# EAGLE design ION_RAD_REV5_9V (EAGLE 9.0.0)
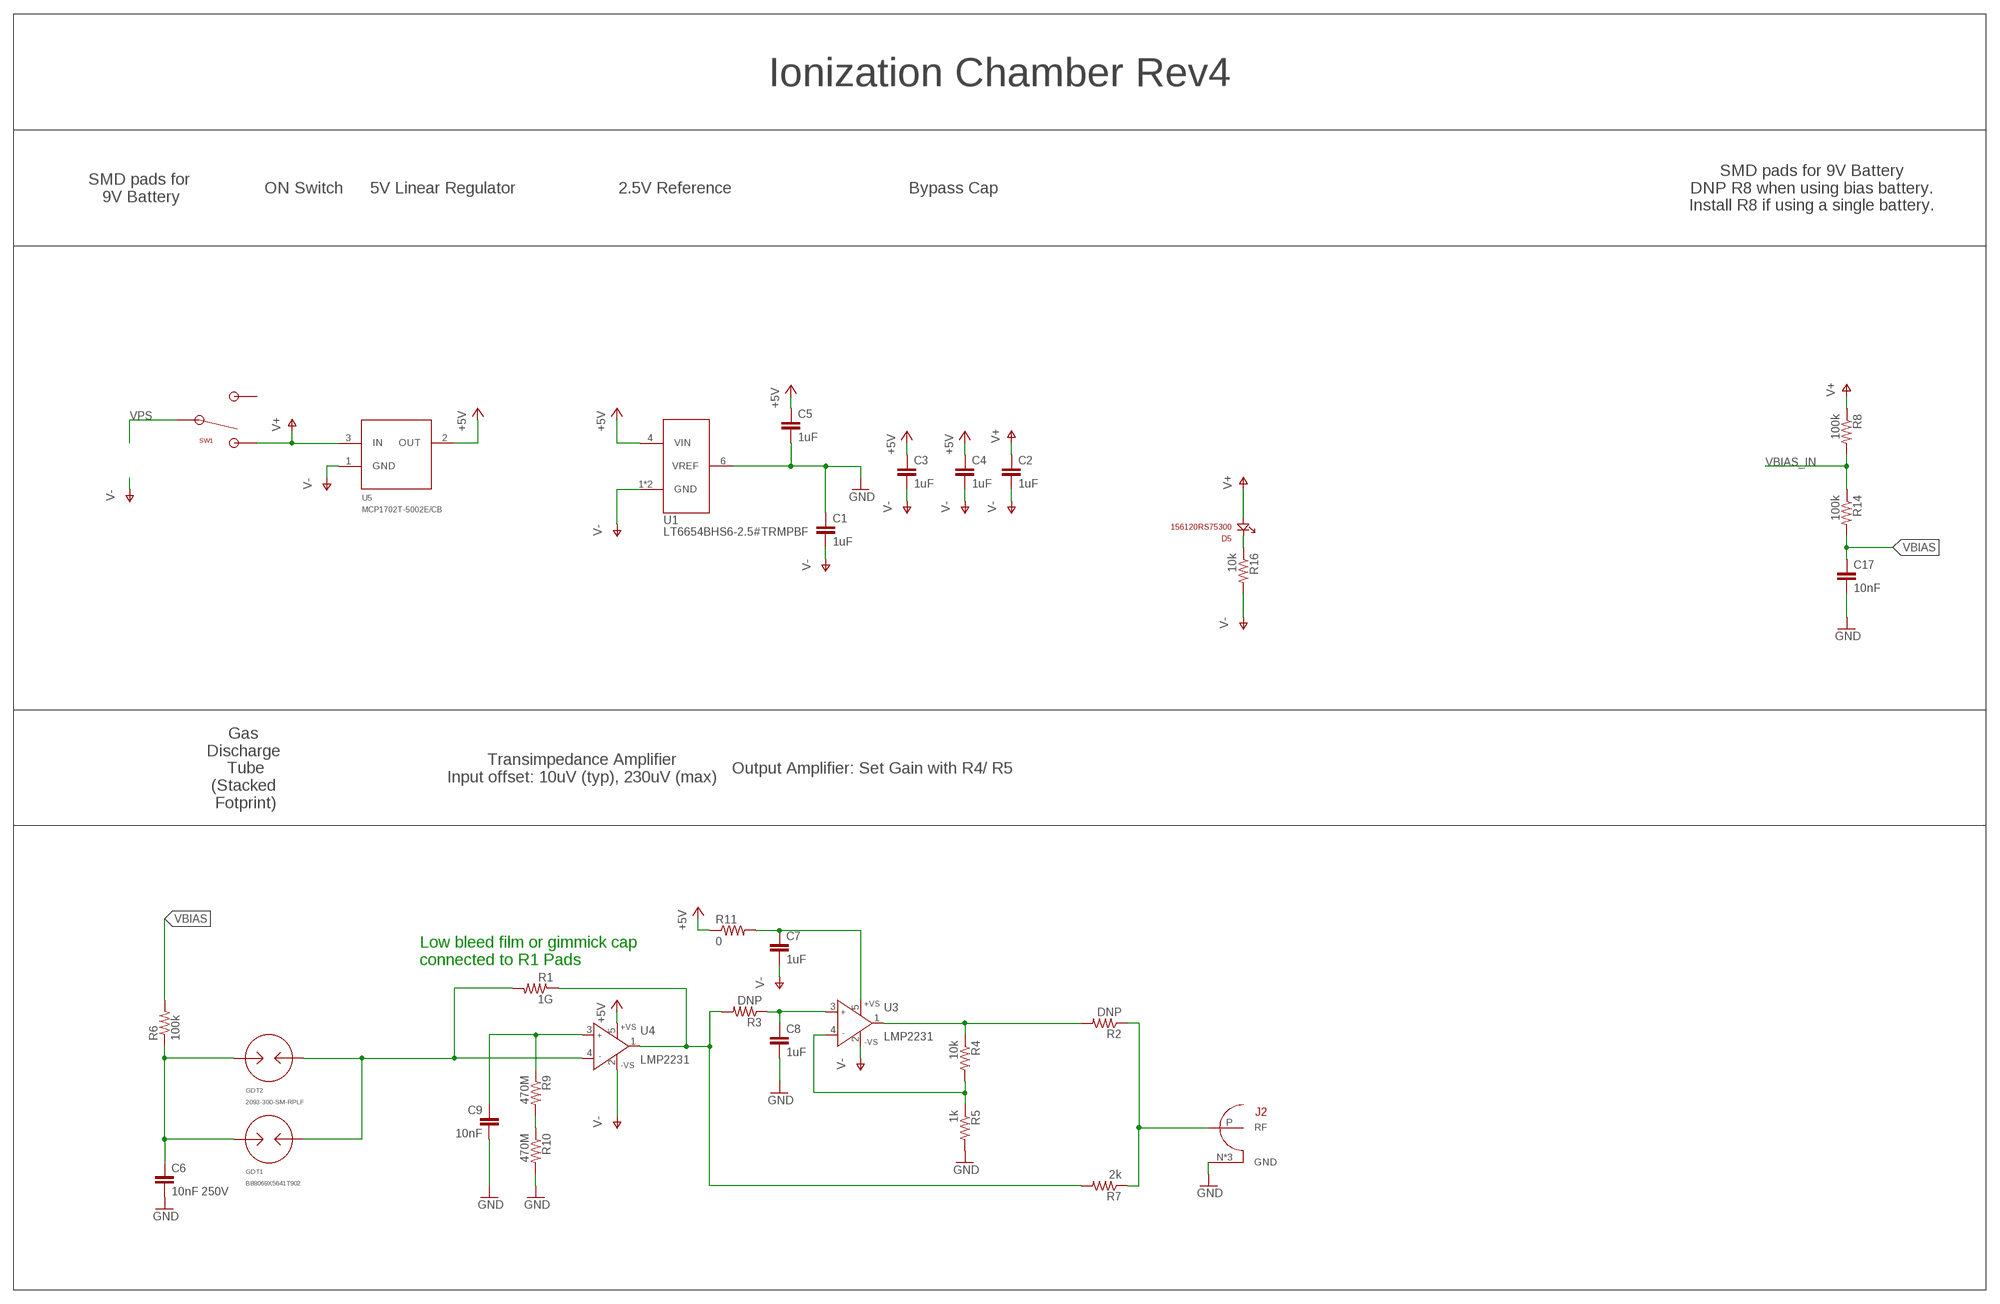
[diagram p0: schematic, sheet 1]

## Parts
C1  1uF  0805_CAPACITOR  [0805]
C2  1uF  0805_CAPACITOR  [0805]
C3  1uF  0805_CAPACITOR  [0805]
C4  1uF  0805_CAPACITOR  [0805]
C5  1uF  0805_CAPACITOR  [0805]
C6  10nF 250V  0805_CAPACITOR  [0805]
C7  1uF  0805_CAPACITOR  [0805]
C8  1uF  0805_CAPACITOR  [0805]
C9  10nF  0805_CAPACITOR  [0805]
C17  10nF  0805_CAPACITOR  [0805]
D5  156120RS75300  [1206_REV]
GDT1  B88069X5641T902  [ES1200XSMD]
GDT2  2093-300-SM-RPLF  [2093-300-SM-RPLF]
J2  0731385033  [0731385033]
R1  1G  MHR0317SA108F70  [MHR0317_SMD]
R2  DNP  0603_RESISTOR  [0603]
R3  DNP  0603_RESISTOR  [0603]
R4  10k  0603_RESISTOR  [0603]
R5  1k  0603_RESISTOR  [0603]
R6  100k  0603_RESISTOR  [0603]
R7  2k  0603_RESISTOR  [0603]
R8  100k  0603_RESISTOR  [0603]
R9  470M  0603_RESISTOR  [0603]
R10  470M  0603_RESISTOR  [0603]
R11  0  0603_RESISTOR  [0603]
R14  100k  0603_RESISTOR  [0603]
R16  10k  0603_RESISTOR  [0603]
SW1  SPDT  100SP1T2B4M6QE  [TOGGLE_RA]
U1  LT6654BHS6-2.5#TRMPBF  [SOT23-6]
U3  LMP2231  [SOT23-5]
U4  LMP2231  [SOT23-5]
U5  MCP1702T-5002E/CB  [SOT23-3_CENTERED]

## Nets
+5V: C3.1 C4.1 C5.1 R11.1 U1.4(VIN) U4.5(+VS) U5.2(OUT)
GND: C1.1 C5.2 C6.2 C8.2 C9.2 C17.2 J2.N(GND) J2.S1(GND) J2.S2(GND) R5.2 R10.2 U1.6(VREF)
INN: GDT1.P$2 GDT2.P$2 R1.P$2 U4.4(IN-)
N$1: C8.1 R3.1 U3.3(IN+)
N$2: R2.2 R4.1 U3.1(OUT)
N$3: R4.2 R5.1 U3.4(IN-)
N$4: C9.1 R9.1 U4.3(IN+)
N$5: J2.P(RF) R2.1 R7.1
N$6: R9.2 R10.1
N$7: C6.1 GDT1.P$1 GDT2.P$1 R6.1
N$10: C7.1 R11.2 U3.5(+VS)
N$19: D5.K R16.1
OUT: R1.P$1 R3.2 R7.2 U4.1(OUT)
V+: C2.1 D5.A R8.1 SW1.3 U5.3(IN)
V-: C1.2 C2.2 C3.2 C4.2 C7.2 R16.2 U1.1(GND) U1.2(GND) U3.2(-VS) U4.2(-VS) U5.1(GND)
VBIAS: C17.1 R6.2 R14.2
VBIAS_IN: R8.2 R14.1
VPS: SW1.2(COM)
Unconnected: SW1.1

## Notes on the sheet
- Ionization Chamber Rev4
- SMD pads for 
  9V Battery
- ON Switch | 5V Linear Regulator | 2.5V Reference | Bypass Cap
- SMD pads for 9V Battery
  DNP R8 when using bias battery.
  Install R8 if using a single battery.
- Gas 
  Discharge 
  Tube
  (Stacked 
  Fotprint)
- Transimpedance Amplifier
  Input offset: 10uV (typ), 230uV (max)
- Output Amplifier: Set Gain with R4/ R5
- Low bleed film or gimmick cap
  connected to R1 Pads

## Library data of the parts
C1-C9 C17 = ruark2:0805_CAPACITOR: NO DEFINED PN
D5 = ruark2:156120RS75300: Red 624nm LED Indication - Discrete 2V 1206 Reverse Mount (3216 Metric); PARTNO: 732-5031-1-ND
GDT1 = ruark2:B88069X5641T902: Gas Discharge Tube 1200V 1000A (1kA) ±15% 2 Pole Surface Mount; PARTNO: 495-76508-1-ND
GDT2 = ruark2:2093-300-SM-RPLF: Gas Discharge Tube 3000V 3000A (3kA) ±20% 2 Pole Surface Mount; PARTNO: 2093-300-SM-RPLFCT-ND
J2 = ruark2:0731385033: BNC Connector Jack, Female Socket 50Ohm Panel Mount, Through Hole, Right Angle Solder; PARTNO: WM5515-ND
R1 = ruark2:MHR0317SA108F70: 1 GOhms ±1% 0.8W Through Hole Resistor Radial High Voltage Thick Film; PARTNO: 490-18223-ND
R2-R11 R14 R16 = ruark2:0603_RESISTOR: 0603 Resistor -- WARNING: NO DEFINED PART NUMBER OR VALUE; VALUE: sel
SW1 = ruark2:100SP1T2B4M6QE: Toggle Switch SPDT Through Hole, Right Angle 5A 120V; PARTNO: EG2362-ND
U1 = ruark2:LT6654BHS6-2.5#TRMPBF: 2.5V Series Voltage Reference IC ±0.1% TSOT-23-6; PARTNO: LT6654BHS6-2.5#TRMPBFCT-ND
U3 U4 = ruark2:LMP2231: General Purpose Amplifier 1 Circuit Rail-to-Rail SOT-23-5, 0.02pA, 10uV
U5 = ruark2:MCP1702T-5002E/CB: Linear Voltage Regulator IC Positive Fixed 1 Output 250mA SOT-23A-3; PARTNO: MCP1702T-5002E/CBCT-ND

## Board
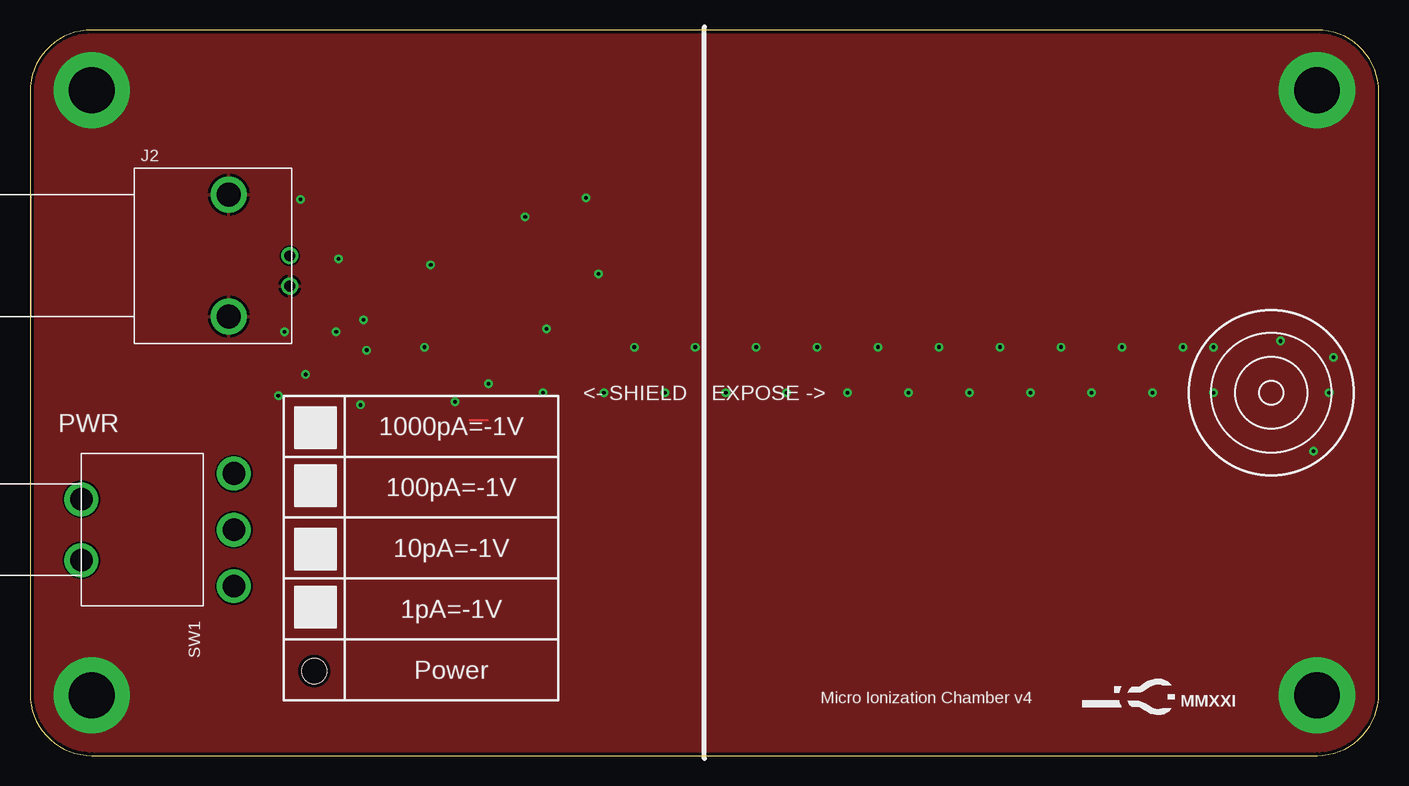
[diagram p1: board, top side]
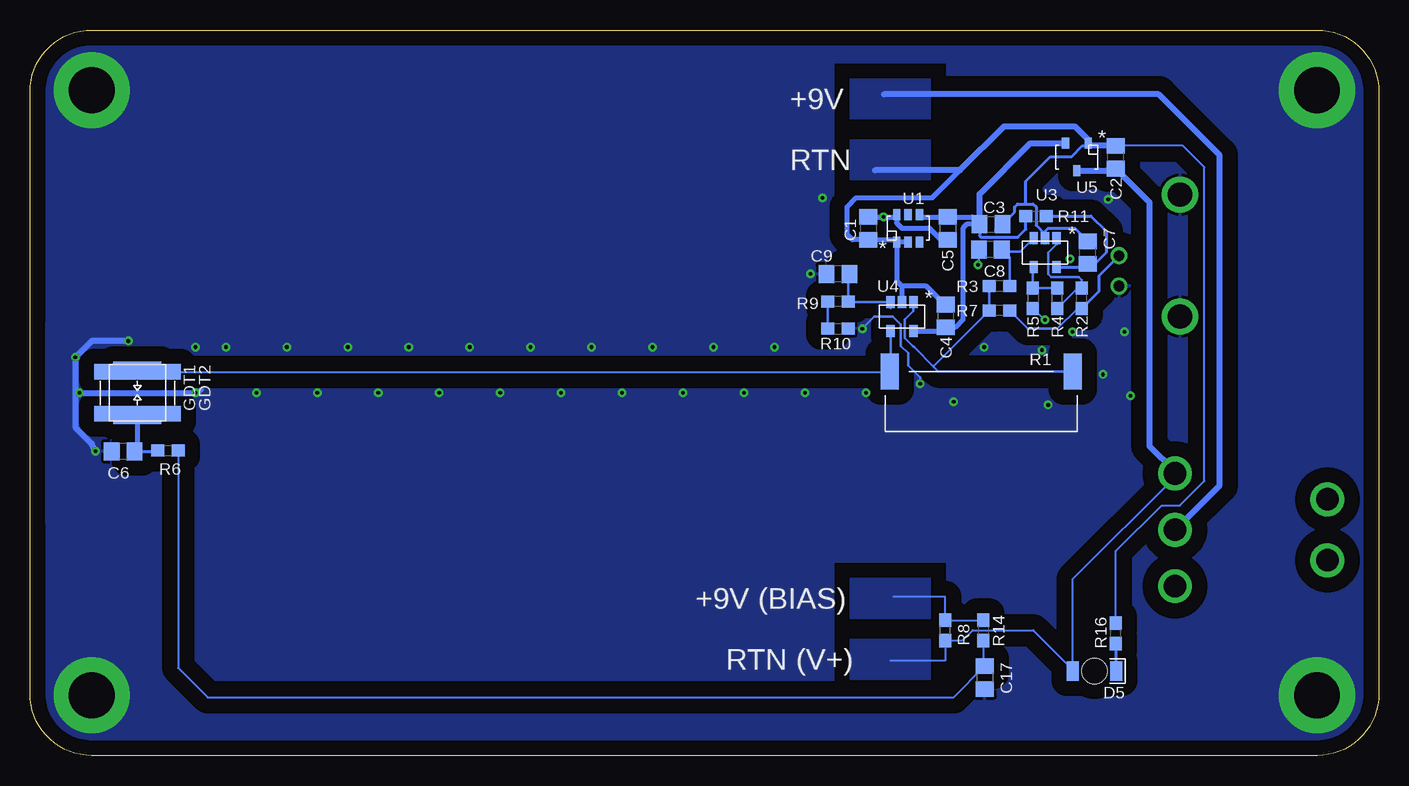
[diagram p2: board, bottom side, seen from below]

Size 112.4 x 60.5 mm. Coordinates in mm from the lower left corner, seen from the top.
Outline: 0,55.35 0,5.15 arc90 5.15,0 107.25,0 arc90 112.4,5.15 112.4,55.35 arc90 107.25,60.5 5.15,60.5 arc90 0,55.35
Copper layers (1*16): Top 0.035mm / dielectric 1.5mm / Bottom 0.035mm
Design rules "default *": minimum track width 6mil, minimum drill 12mil, track to track 6mil, track to pad 6mil, pad to pad 6mil, via to via 6mil, smd to smd 6mil, copper to edge 0.3mm, drill to drill 6mil, minimum pad ring 10mil, minimum via ring 8mil, stop-mask expansion 4mil, vias tented up to drill 12mil, thermal gap 10mil

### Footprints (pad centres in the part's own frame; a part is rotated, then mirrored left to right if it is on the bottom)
0805 = smd 1.3 x 1.5: 1 -0.95,0; 2 0.95,0
1206_REV = smd 1 x 1.6: A -1.8,0; K 1.8,0 | hole 2.1: 0,0
ES1200XSMD = smd 1.25 x 4: P$1 -1.975,0; P$2 1.975,0
2093-300-SM-RPLF = smd 1.3 x 7.2: P$1 -1.75,0; P$2 1.75,0
0731385033 = drill 0.889: N -2.54,-5.08; P 0,-5.08 | drill 2.007: S1 -5.08,0; S2 5.08,0
MHR0317_SMD = smd 1.5 x 3: P$1 -7.62,0; P$2 7.62,0
0603 = smd 1.1 x 1: 1 -0.85,0; 2 0.85,0
TOGGLE_RA = drill 1.88: 1 4.699,12.7; 2 0,12.7; 3 -4.699,12.7; P$4 -2.54,0; P$5 2.54,0
SOT23-6 = smd 0.6 x 0.9: 1 -0.95,-1.15; 2 0,-1.15; 3 0.95,-1.15; 4 0.95,1.15; 5 0,1.15; 6 -0.95,1.15
SOT23-5 = smd 0.7 x 1: 1 0.95,1.2; 2 0,1.2; 3 -0.95,1.2; 4 -0.95,-1.2; 5 0.95,-1.2
SOT23-3_CENTERED = smd 0.6 x 0.9: 1 -0.95,-1.15; 2 0.95,-1.15; 3 0,1.15

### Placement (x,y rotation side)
C1  42.53,43.97 270 bottom
C2  21.91,49.88 90 bottom
C3  32.32,44.3 0 bottom
C4  36.07,36.65 90 bottom
C5  35.93,43.97 270 bottom
C6  104.63,25.36 180 bottom
C7  24.25,41.93 90 bottom
C8  32.37,42.19 180 bottom
C9  45.07,40.16 180 bottom
C17  32.83,6.5 270 bottom
D5  23.69,7.03 0 bottom
GDT1  103.44,30.25 90 bottom
GDT2  103.44,30.25 90 bottom
J2  16.57,41.68 90 top
R1  33.14,32.03 180 bottom
R2  24.75,38.12 90 bottom
R3  31.61,39.14 180 bottom
R4  26.79,38.12 90 bottom
R5  28.82,38.12 270 bottom
R6  100.9,25.42 0 bottom
R7  31.61,37.11 180 bottom
R8  36.13,10.44 90 bottom
R9  45.07,37.87 180 bottom
R10  45.07,35.58 0 bottom
R11  28.56,44.98 0 bottom
R14  32.96,10.44 270 bottom
R16  21.91,10.18 90 bottom
SW1  4.28,18.82 270 top
U1  39.23,43.97 0 bottom
U3  27.8,41.93 0 bottom
U4  39.74,36.6 0 bottom
U5  25.16,49.91 180 bottom

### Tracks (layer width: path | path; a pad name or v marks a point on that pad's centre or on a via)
+5V
  Bottom 0.254: C3.1 33.27,43.34 33.15,43.22 30.08,43.22 29.42,43.88 R11.1
  Bottom 0.406: 33.89,44.92 C5.1 38.08,44.92 U1.4 | 33.89,44.92 C3.1 34.33,44.3 34.66,43.97 34.66,36.35 35.31,35.7 C4.1 36.63,35.4 U4.5 | 33.9,44.91 33.89,44.92
  Bottom 0.508: C3.1 33.27,46.83 29.04,51.06 U5.2
GND  (via drill 0.3, 3.81 pad 6.35)
  Top 0.152: 36.64,27.96 38.17,27.96
  Bottom 0.203: R5.2 27.89,36.35 v27.8,36.35 | C8.2 33.33,40.98 v33.39,40.92 | v43.04,35.58 42.03,36.6 40.5,36.6 39.84,35.94 39.84,34.16 39.23,33.55 39.23,32.54 38.22,31.52 v38.22,31.01
  Bottom 0.406: 98.36,30.25 98.11,30.5 | C1.1 v41.27,44.92 40.38,44.92 U1.6 40.18,44.41 39.74,43.97 37.45,43.97 36.51,43.02 C5.2
  Bottom 0.508: v104.21,34.57 107.25,34.57 v108.63,33.2 108.63,30.25 | 108.63,30.25 108.63,27.35 107.25,25.98 v106.95,25.37 | 108.63,30.25 v108.27,30.25 v98.62,30.25
  other vias: 5.15,55.48 5.15,5.02 107.25,55.48 107.25,5.02 98.62,34.06 28.06,33.81 22.55,46.38 25.72,41.43 32.88,34.06 25.52,35.33 22.98,31.77 20.69,30 47.36,40.16 46.34,46.51 27.55,29.23 21.2,35.33 35.42,29.49 93.54,30.25 88.46,30.25 96.08,34.06 91,34.06 85.92,34.06 83.38,30.25 78.3,30.25 80.84,34.06 75.76,34.06 70.68,34.06 65.6,34.06 60.52,34.06 55.44,34.06 50.36,34.06 73.22,30.25 68.14,30.25 63.06,30.25 57.98,30.25 52.9,30.25 47.82,30.25 42.74,30.25
  pour Top: 0.2,54.25 0.2,55.1 arc-90 5.35,60.25 107.05,60.25 arc-90 112.2,55.1 112.2,5.4 arc-90 107.05,0.25 5.35,0.25 arc-90 0.2,5.4
  pour Bottom (isolate 1.27, rank 4): 0.2,54.25 0.2,55.1 arc-90 5.35,60.25 107.05,60.25 arc-90 112.2,55.1 112.2,5.4 arc-90 107.05,0.25 5.35,0.25 arc-90 0.2,5.4
  pour Bottom: 109.84,33.45 109.84,36.04 111.06,36.04 111.06,19.43 109.84,19.43
INN
  Bottom 0.152: GDT2.P$2 40.79,32 R1.P$2 | 103.64,32.19 GDT2.P$2 | GDT2.P$2 GDT1.P$2
  Bottom 0.203: U4.4 40.69,32.09 R1.P$2
N$1
  Bottom 0.203: R3.1 30.76,41.53 31.27,42.03 | 31.27,42.03 C8.1 | U3.3 29.86,42.03 31.27,42.03
N$2
  Bottom 0.203: R4.1 25.09,38.97 R2.2 24.76,39.65 25.01,39.9 27.3,39.9 27.55,40.16 27.55,41.93 26.85,42.63 U3.1
N$3
  Bottom 0.203: R4.2 R5.1 28.82,40.67 U3.4
N$4
  Bottom 0.203: 40.69,37.3 U4.3 44.16,37.8 R9.1 44.23,40.06 C9.1
N$5
  Bottom 0.203: R7.1 29.24,35.58 26.79,35.58 25.1,37.27 R2.1 24.59,37.11
  Bottom 0.254: R2.1 23.31,38.72 23.31,40.02 J2.P
N$6
  Bottom 0.203: R9.2 R10.1
N$7
  Bottom 0.152: GDT1.P$1 GDT2.P$1
  Bottom 0.254: C6.1 101.82,25.36 R6.1
  Bottom 0.406: GDT2.P$1 103.44,25.6 C6.1
N$10
  Bottom 0.254: R11.2 23.99,44.98 22.72,43.71 22.72,41.93 23.67,40.98 C7.1 25.01,40.73 U3.5
N$19
  Bottom 0.254: D5.K 21.89,9.31 R16.1
OUT
  Bottom 0.203: U4.1 38.79,37.04 39.49,36.35 39.49,34.82 38.83,34.16 38.73,34.06 37.07,32.41 | R1.P$1 36.69,32.03 37.07,32.41 | 32.52,37.32 R7.2 | R7.2 37.07,32.5 37.07,32.41 | R7.2 R3.2
V+
  Bottom 0.152: 17.14,23.52 16.98,23.67 16.98,23.24 25.49,14.73 25.49,7.14 | D5.A 25.49,7.14 | 40.71,7.9 36.13,7.9 R8.1 34.7,9.59 33.85,10.44 28.79,10.44 25.49,7.14
  Bottom 0.254: D5.A 25.47,7.06
  Bottom 0.508: U5.3 22.59,48.76 C2.1 19.12,46.14 19.12,25.8 16.98,23.67
  Bottom 1.016: 16.98,23.67 SW1.3
  pour Bottom: 44.01,9.68 37.4,9.68 37.4,6.37 44.01,6.37
V-
  Bottom 0.152: R16.2 21.91,17.04 18.1,20.85 16.58,20.85 14.54,22.88 14.54,49.05 16.33,50.83 C2.2
  Bottom 0.254: C3.2 30.34,45.33 30.34,45.74 30.09,46 29.4,46 | 29.4,46 28.82,46 28.57,45.74 28.57,44.22 27.8,43.46 U3.2 27.8,43.71 27.55,43.97 25.33,43.97 C7.2 | 29.4,46 29.4,47.9 27.37,49.94 25.59,49.94 24.69,50.83 23.99,50.83
  Bottom 0.406: 31.87,43.8 C3.2 31.11,44.57 | U1.2 U1.1 | U1.1 40.38,43.02 C1.2 43.87,43.02 44.31,43.46 44.31,45.74 43.55,46.51 37.2,46.51 34.92,48.79 | U1.1 40.18,39.58 39.74,39.14 | 39.74,39.14 U4.2 | C4.2 36.58,38.01 37.71,39.14 39.74,39.14
  Bottom 0.508: C2.2 23.99,50.83 U5.1 24.21,51.35 25.34,52.48 31.23,52.48 34.92,48.79 41.98,48.79
  pour Bottom: 44.01,51.33 37.4,51.33 37.4,48.03 44.01,48.03
VBIAS
  Bottom 0.152: R6.2 100.05,7.3 97.6,4.85 35.43,4.85 32.86,7.42 | 32.86,7.42 C17.1 | R14.2 32.96,7.52 32.86,7.42
VBIAS_IN
  Bottom 0.152: 40.45,13.23 36.13,13.23 R8.2 R14.1
  pour Bottom: 44.01,14.76 37.4,14.76 37.4,11.45 44.01,11.45
VPS
  Bottom 0.508: SW1.2 13.27,22.53 13.27,50.06 18.35,55.14 41.21,55.14
  pour Bottom: 44.01,56.41 37.4,56.41 37.4,53.11 44.01,53.11

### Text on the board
tPlace: Micro Ionization Chamber v4 | MMXXI
bPlace: +9V | RTN | +9V (BIAS) | RTN (V+)
tNames: <- SHIELD EXPOSE -> | PWR | 1000pA=-1V | 100pA=-1V | 10pA=-1V | 1pA=-1V | Power
tStop: 037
